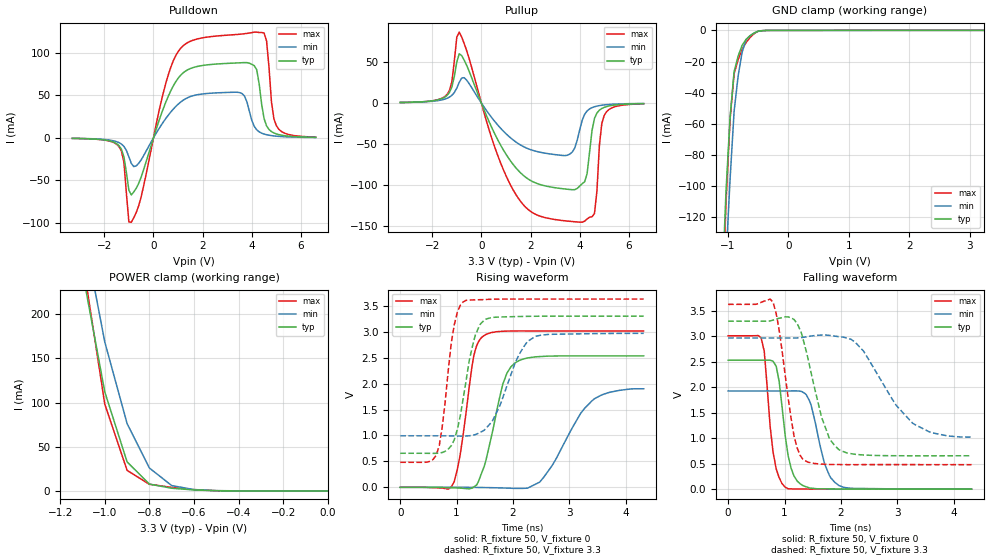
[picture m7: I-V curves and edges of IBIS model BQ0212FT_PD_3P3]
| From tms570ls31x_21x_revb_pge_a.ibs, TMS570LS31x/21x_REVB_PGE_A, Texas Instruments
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|   Model Cell BQ0212FT_PD_3P3
|BQ0212FT_PD_3P3
[Model]   BQ0212FT_PD_3P3
Model_type   I/O
Polarity   Non-Inverting
Enable   Active-Low
Vinl =  1.15
Vinh =  1.55
Cref =  15.0001pF
Rref =  101.0000M
Vref =  0V
Vmeas =  1.65
C_comp   1.2p   1.2p   1.2p
[Model Spec]
Vinl   1.15   1.02   1.28
Vinh   1.55   1.45   1.65
[Temperature Range]   25   155   -40
[Voltage Range]   3.3   2.97   3.63
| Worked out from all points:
|   slope of the pulldown table from 0 to 0.495 V, typ, clamps not added: 11.9 ohm
|   slope of the pullup table from 0 to 0.495 V, typ, clamps not added: 14.3 ohm
|   GND clamp passes 1 mA (typ) near -0.53 V on its own axis
|   POWER clamp passes 1 mA (typ) near -0.59 V on its own axis
|   rising waveform, R_fixture 50, V_fixture 0: 20-80 % time 316ps typ, 599ps min, 226ps max; typ from 0 V to 2.53 V
|   rising waveform, R_fixture 50, V_fixture 3.3: 20-80 % time 266ps typ, 432ps min, 201ps max; typ from 0.657 V to 3.3 V
|   falling waveform, R_fixture 50, V_fixture 0: 20-80 % time 182ps typ, 258ps min, 155ps max; typ from 2.53 V to 0 V
|   falling waveform, R_fixture 50, V_fixture 3.3: 20-80 % time 362ps typ, 700ps min, 238ps max; typ from 3.3 V to 0.656 V
[POWER_clamp]
|   voltage   I(typ)   I(min)   I(max)
-3.3V     4.054A     4.63A      4.887A
-1.1V     248.3mA    301mA      262.7mA
-1.067V   202.9mA    256.9mA    207.9mA
-1.033V   157.5mA    212.7mA    153.1mA
-1V       112.1mA    168.6mA    98.31mA
-900mV    32.89mA    76.23mA    23.26mA
-800mV    7.724mA    25.95mA    7.513mA
-700mV    3.052mA    6.046mA    4.028mA
-600mV    1.107mA    1.536mA    1.463mA
-500mV    206.8uA    377.5uA    241.6uA
0V        19.75uA    8.57uA     38.26uA
[Pulldown]
|   voltage   I(typ)   I(min)   I(max)
-3.3V     -593uA     -522.6uA   -580.3uA
-1.4V     -9.188mA   -5.565mA   -10.35mA
-1.2V     -22.55mA   -10.08mA   -29.13mA
-1V       -61.66mA   -22.23mA   -99.07mA
-900mV    -67.21mA   -30.1mA    -99.29mA
1V        70.16mA    39.61mA    101.5mA
3.5V      88.44mA    53.41mA    122.1mA
4.2V      80.27mA    9.542mA    124.6mA
4.6V      14.18mA    3.749mA    114.2mA
4.8V      7.418mA    2.695mA    42.04mA
5V        4.687mA    2.03mA     14.29mA
6.6V      680.4uA    493.7uA    947.4uA
[Pullup]
|   voltage   I(typ)   I(min)   I(max)
-3.3V     671.9uA    618.2uA    613.1uA
-1.4V     9.171mA    5.687mA    10.35mA
-900mV    59.98mA    25.21mA    86.36mA
600mV     -40.93mA   -24.46mA   -58.45mA
1.4V      -78.76mA   -47.34mA   -111.2mA
3.5V      -105mA     -63.56mA   -143.7mA
4.1V      -98.17mA   -21.1mA    -145.1mA
4.3V      -85.91mA   -9.61mA    -141.1mA
4.6V      -18.69mA   -4.516mA   -134.6mA
4.8V      -8.691mA   -3.128mA   -51.49mA
5V        -5.242mA   -2.297mA   -14.81mA
6.6V      -711.8uA   -541.3uA   -921.2uA
[GND_clamp]
|   voltage   I(typ)   I(min)   I(max)
-3.3V     -3.25A     -2.875A    -4.945A
-1.1V     -166.9mA   -205mA     -187mA
-1.033V   -102.8mA   -146.7mA   -110.1mA
-966.7mV  -55.96mA   -95.69mA   -57.02mA
-900mV    -26.55mA   -52.03mA   -27.8mA
-833.3mV  -16.5mA    -29.28mA   -18.78mA
-766.7mV  -9.547mA   -13.91mA   -12.08mA
-700mV    -5.701mA   -5.927mA   -7.726mA
-566.7mV  -1.578mA   -1.635mA   -2.073mA
-500mV    -412.7uA   -599.4uA   -476.8uA
-366.7mV  -26.33uA   -63.11uA   -29.79uA
3.233V    19.75uA    12.65uA    38.26uA
[Ramp]
| variable   typ   min   max
dV/dt_f   1.638063/0.3730528n   1.223184/0.7332278n   1.953359/0.245381n
dV/dt_r   1.540087/0.3185134n   1.172095/0.6252384n   1.831372/0.2272384n
R_load = 50
[Rising Waveform]
R_fixture = 50
V_fixture = 0
V_fixture_min = 0
V_fixture_max = 0
|   time   V(typ)   V(min)   V(max)
0s        -4.808uV   -2.599uV   -6.607uV
956ps     -9.903mV   198.8uV    104.8mV
1.064ns   -15.37mV   128.5uV    634.3mV
1.304ns   7.129mV    -1.953mV   2.535V
1.492ns   413.3mV    -4.659mV   2.929V
1.82ns    1.992V     -12.78mV   3.009V
2.036ns   2.4V       -21.31mV   3.015V
2.472ns   2.521V     99.74mV    3.014V
3.444ns   2.534V     1.707V     3.014V
4.316ns   2.533V     1.9V       3.014V
[Rising Waveform]
R_fixture = 50
V_fixture = 3.3
V_fixture_min = 2.97
V_fixture_max = 3.63
|   time   V(typ)   V(min)   V(max)
0s        656.5mV    993.1mV    482.3mV
640ps     655.5mV    993.2mV    623.1mV
744ps     670.9mV    993mV      1.161V
956ps     910.9mV    990.2mV    3.124V
1.116ns   1.71V      987.8mV    3.575V
1.332ns   2.935V     1.016V     3.614V
1.52ns    3.243V     1.138V     3.622V
2.108ns   3.293V     2.561V     3.63V
2.4ns     3.298V     2.91V      3.63V
4.316ns   3.3V       2.968V     3.63V
[Falling Waveform]
R_fixture = 50
V_fixture = 0
V_fixture_min = 0
V_fixture_max = 0
|   time   V(typ)   V(min)   V(max)
0s        2.533V     1.93V      3.014V
584ps     2.533V     1.93V      2.974V
640ps     2.533V     1.93V      2.709V
852ps     2.414V     1.93V      398.3mV
1.012ns   1.045V     1.929V     39.11mV
1.168ns   258.4mV    1.93V      4.035mV
1.384ns   46.16mV    1.858V     2.57mV
1.712ns   5.204mV    493.8mV    575.6uV
1.964ns   2.891mV    71.92mV    316.6uV
4.316ns   95.04uV    836.3uV    2.631uV
[Falling Waveform]
R_fixture = 50
V_fixture = 3.3
V_fixture_min = 2.97
V_fixture_max = 3.63
|   time   V(typ)   V(min)   V(max)
0s        3.3V       2.97V      3.63V
796ps     3.321V     2.97V      3.673V
904ps     3.358V     2.97V      3.126V
1.168ns   3.333V     2.969V     1.044V
1.332ns   2.931V     2.983V     578.1mV
1.656ns   1.416V     3.027V     492.6mV
1.964ns   775.5mV    2.995V     483mV
2.4ns     671.5mV    2.713V     482.5mV
3.268ns   655.6mV    1.298V     482.4mV
4.316ns   656.4mV    1.023V     482.3mV
